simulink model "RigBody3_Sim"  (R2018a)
settings: Solver=ode3  StartTime=0.0  StopTime=5000  FixedStep=Tsr  RelTol=1e-3  EnableMultiTasking=on
InitFcn:
  | run
StopFcn:
  | pl
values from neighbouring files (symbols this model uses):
  d2r = pi/180    (= 0.0174532925199)    [orbitic.m]    (also in Quan.m; run.m; runf.m)
  Int_IC = [qti', 0 0, h0i(1:3)', 0 0, wr0, Vec0'*M0, Pec0']    [run.m]
  Kq1 = I22*ww^2 - 3*wo2*(I11-I33)    [run.m]
  Kq2 = 2*I22*zet*ww    [run.m]
  Kqi = 0.0005    [run.m]
  Kr1 = (0.1*I11*I33*zet^2/Hy0) - sqrt( ((0.01^zet^4*I11^2*I33^2)/Hy0^2)+(4*I11*I33*zet^2) )    [run.m]
  Kr2 = 0.05*Kr1    [run.m]
  Kr3 = 0.04*zet*(Kr2-Hy0) * sqrt(abs(Hy0/(I11*I33)))    [run.m]
  nt = 7    [run.m]    (also in runf.m)
  r2d = 180/pi    (= 57.2957795131)    [pl.m]    (also in pl2.m; run.m; plf.m; runf.m)
  Tmax = 0.05    [run.m]
  Tsr = 0.1    [run.m]
  wo = 0.00113    [run.m]
undefined symbols (not defined in the file or in its folder): DiscIntNeverNeededParam, Mode_Switch, Phase_Plane, RW_Steering, Vehi_3B3W
libraries: simulink x4

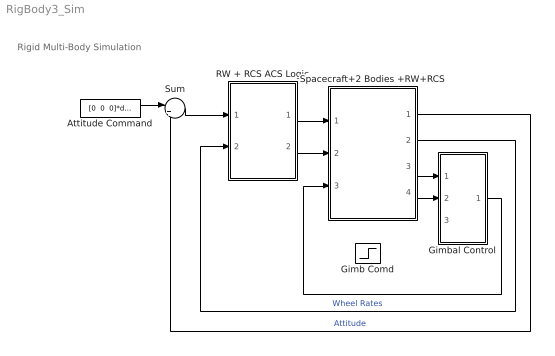
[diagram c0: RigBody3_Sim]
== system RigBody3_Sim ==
  note: Rigid Multi-Body Simulation
  Attitude Command : Constant  Value="[0  0  0]*d2r"
  Gimb Comd : Step  Time=[1, 1]*2000  After=[5, 5]*d2r  SampleTime=0
  Gimbal Control : Subsystem
  RW + RCS ACS Logic : Subsystem
  Spacecraft+2 Bodies +RW+RCS : Subsystem
  Sum : Sum  Inputs=|+-
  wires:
  Spacecraft+2 Bodies +RW+RCS/2(Wrw) -> RW + RCS ACS Logic/2(wr(i))  "Wheel Rates"
  Attitude Command/1 -> Sum/1
  Spacecraft+2 Bodies +RW+RCS/1(att) -> Sum/2  "Attitude"
  Sum/1 -> RW + RCS ACS Logic/1(atter)
  RW + RCS ACS Logic/2(Trwi) -> Spacecraft+2 Bodies +RW+RCS/2(Trw)
  RW + RCS ACS Logic/1(Frcs) -> Spacecraft+2 Bodies +RW+RCS/1(Fjets)
  Spacecraft+2 Bodies +RW+RCS/4(Gmb-dot) -> Gimbal Control/2(Grat)
  Spacecraft+2 Bodies +RW+RCS/3(gimb) -> Gimbal Control/1(Gimb)
  Gimbal Control/1(Trq) -> Spacecraft+2 Bodies +RW+RCS/3(Tgimb)

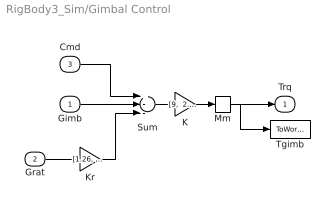
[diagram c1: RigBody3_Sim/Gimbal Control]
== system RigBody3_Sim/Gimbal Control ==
  Gimb : Inport
  Grat : Inport  Port=2
  Cmd : Inport  Port=3
  K : Gain  Gain="[9,  2.85]"
  Kr : Gain  Gain="[1.26,  1.14]"
  Mm : Memory  InheritSampleTime=on
  Sum : Sum  Inputs=+--
  Tgimb : ToWorkspace  VariableName=Tgimb  SampleTime=-1
  Trq : Outport
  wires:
  Sum/1 -> K/1
  Gimb/1 -> Sum/2
  Grat/1 -> Kr/1
  K/1 -> Mm/1
  Kr/1 -> Sum/3
  Cmd/1 -> Sum/1
  Mm/1 -> Trq/1, Tgimb/1

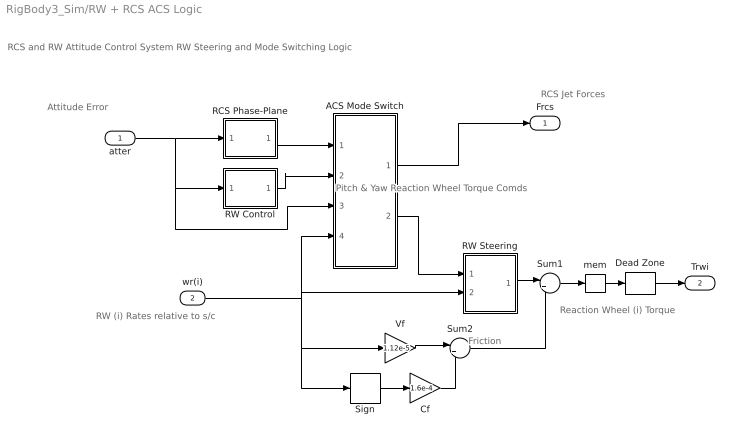
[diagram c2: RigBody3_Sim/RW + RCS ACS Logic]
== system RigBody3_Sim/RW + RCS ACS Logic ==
  note: RCS Jet Forces
  note: RW (i) Rates relative to s/c
  note: Attitude Error
  note: Pitch & Yaw Reaction Wheel Torque Comds
  note: Friction
  note: Reaction Wheel (i) Torque
  note: RCS and RW Attitude Control System RW Steering and Mode Switching Logic
  atter : Inport
  wr(i) : Inport  Port=2
  ACS Mode Switch : Subsystem
  Cf : Gain  Gain=1.6e-4
  Dead Zone : DeadZone  LowerValue=-[1, 1, 1]*Tmax/1000  UpperValue=[1 1 1]*Tmax/1000
  RCS Phase-Plane : Subsystem
  RW Control : Subsystem
  RW Steering : Subsystem
  Sign : Signum
  Sum1 : Sum  Inputs=|+-
  Sum2 : Sum  Inputs=|++
  Vf : Gain  Gain=1.12e-5
  mem : Memory  InheritSampleTime=on
  Frcs : Outport
  Trwi : Outport  Port=2
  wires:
  atter/1 -> RCS Phase-Plane/1(atter), ACS Mode Switch/3(atter), RW Control/1(atti)
  RW Control/1(Tc) -> ACS Mode Switch/2(Trw)
  RCS Phase-Plane/1(f(nt)) -> ACS Mode Switch/1(Frcs)
  ACS Mode Switch/2(" Trw") -> RW Steering/1(Trwc)
  ACS Mode Switch/1(" Frcs") -> Frcs/1
  wr(i)/1 -> Vf/1, Sign/1, RW Steering/2(wr(1)), ACS Mode Switch/4(wr(i))
  Sum2/1 -> Sum1/2
  Sign/1 -> Cf/1
  Vf/1 -> Sum2/1
  Cf/1 -> Sum2/2
  RW Steering/1(Twi) -> Sum1/1
  Sum1/1 -> mem/1
  mem/1 -> Dead Zone/1
  Dead Zone/1 -> Trwi/1

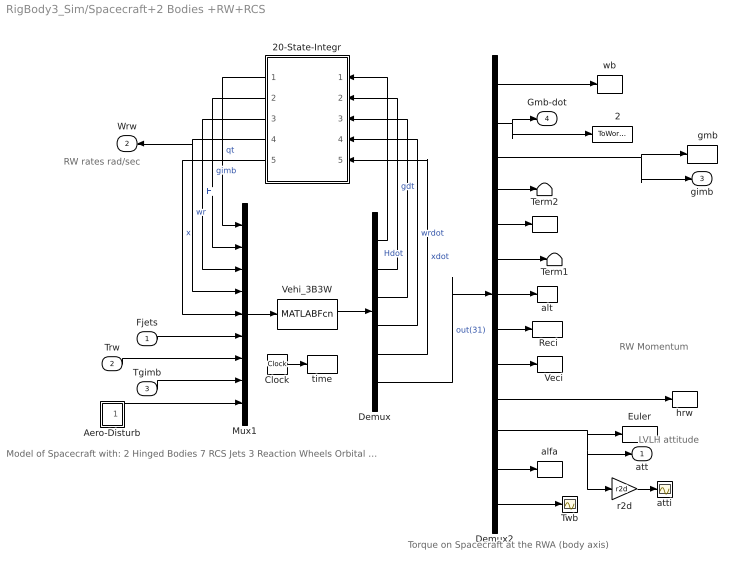
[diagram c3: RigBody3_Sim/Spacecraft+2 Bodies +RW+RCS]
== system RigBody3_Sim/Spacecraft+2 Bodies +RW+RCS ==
  note: RW rates rad/sec
  note: RW Momentum
  note: Model of Spacecraft with: 2 Hinged Bodies 7 RCS Jets 3 Reaction Wheels Orbital Dynamics
  note: LVLH attitude
  note: Torque on Spacecraft at the RWA (body axis)
  Fjets : Inport
  Trw : Inport  Port=2
  Tgimb : Inport  Port=3
  "    " : ToWorkspace  VariableName=hsys  SampleTime=-1
  "    2" : ToWorkspace  VariableName=Gimdot  SampleTime=-1
  "    gmb" : ToWorkspace  VariableName=Gimb  SampleTime=-1
  "   Veci" : ToWorkspace  VariableName=Veci  SampleTime=-1
  "  Reci " : ToWorkspace  VariableName=Reci  SampleTime=-1
  20-State-Integr : Subsystem
  Aero-Disturb : Subsystem
  Clock : Clock
  Demux : Demux  Outputs="[4,2,5,3,6,  31]"
  Demux2 : Demux  Outputs=[3,2,2,1, 3,2, 1,3,3,3,3, 2,3]
  Euler : ToWorkspace  VariableName=Euler  SampleTime=-1
  Mux1 : Mux  Inputs="[4,2,5,3,6,  nt,3,2,3]"
  Term1 : Terminator
  Term2 : Terminator
  Twb : Scope
  Vehi_3B3W : MATLABFcn  MATLABFcn=Vehi_3B3W( u(1:20), u(21:20+nt), u(21+nt:23+nt), u(24+nt:25+nt), u(26+nt:28+nt) )  OutputDimensions=51
  alfa : ToWorkspace  VariableName=alfa  SampleTime=-1
  alt : ToWorkspace  VariableName=alt  SampleTime=-1
  atti : Scope
  hrw : ToWorkspace  VariableName=hrw  SampleTime=-1
  r2d : Gain  Gain=r2d
  time : ToWorkspace  VariableName=time  SampleTime=-1
  wb : ToWorkspace  VariableName=wb  SampleTime=-1
  att : Outport
  Wrw : Outport  Port=2
  gimb : Outport  Port=3
  Gmb-dot : Outport  Port=4
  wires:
  Demux2/9 -> "   Veci"/1
  Vehi_3B3W/1 -> Demux/1
  20-State-Integr/1(qt) -> Mux1/1  "qt"
  20-State-Integr/2(gimb) -> Mux1/2  "gimb"
  20-State-Integr/3(H) -> Mux1/3  "H"
  20-State-Integr/4(wr) -> Wrw/1, Mux1/4  "wr"
  20-State-Integr/5(x) -> Mux1/5  "x"
  Demux/6 -> Demux2/1  "out(31)"
  Demux/1 -> 20-State-Integr/1(qdot)
  Demux/2 -> 20-State-Integr/2(gmbdot)  "gdt"
  Demux/3 -> 20-State-Integr/3(Hdot)  "Hdot"
  Demux/4 -> 20-State-Integr/4(wrdor)  "wrdot"
  Demux/5 -> 20-State-Integr/5(xdot)  "xdot"
  Demux2/12 -> alfa/1
  Demux2/11 -> Euler/1, att/1, r2d/1
  Demux2/10 -> hrw/1
  Demux2/8 -> "  Reci "/1
  Demux2/7 -> alt/1
  Demux2/5 -> "    "/1
  Demux2/6 -> Term1/1
  Demux2/1 -> wb/1
  Demux2/4 -> Term2/1
  Demux2/2 -> Gmb-dot/1, "    2"/1
  Demux2/3 -> gimb/1, "    gmb"/1
  Clock/1 -> time/1
  Tgimb/1 -> Mux1/8
  Aero-Disturb/1(Td) -> Mux1/9
  Trw/1 -> Mux1/7
  Fjets/1 -> Mux1/6
  Mux1/1 -> Vehi_3B3W/1
  r2d/1 -> atti/1
  Demux2/13 -> Twb/1

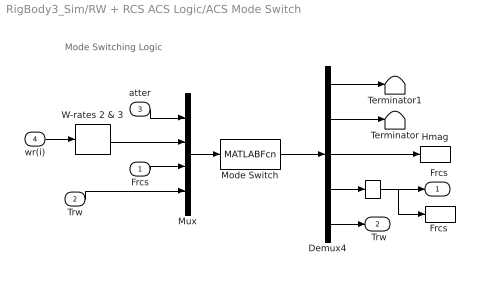
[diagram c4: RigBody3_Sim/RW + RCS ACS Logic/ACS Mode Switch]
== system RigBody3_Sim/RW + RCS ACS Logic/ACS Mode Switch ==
  note: Mode Switching Logic
  Frcs : Inport
  Trw : Inport  Port=2
  atter : Inport  Port=3
  wr(i) : Inport  Port=4
  "   " : Memory
  Demux4 : Demux  Outputs="[1 1 1 nt  2]"
  "Frcs " : ToWorkspace  VariableName=Frcs  SampleTime=-1
  Hmag : ToWorkspace  VariableName=Hmag  SampleTime=-1
  Mode Switch : MATLABFcn  MATLABFcn=Mode_Switch( u(1:3), u(4:5), u(6:5+nt), u(6+nt:7+nt) )  OutputDimensions=3+nt+2
  Mux : Mux  Inputs="[3  2  nt 2]"
  Terminator : Terminator
  Terminator1 : Terminator
  W-rates 2 & 3 : Selector  InputPortWidth=3  IndexOptions=Index vector (dialog)  Indices="[2  3]"  OutputSizes=1
  " Frcs" : Outport
  " Trw" : Outport  Port=2
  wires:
  Demux4/3 -> Hmag/1
  Demux4/2 -> Terminator/1
  Demux4/1 -> Terminator1/1
  W-rates 2 & 3/1 -> Mux/2
  "   "/1 -> " Frcs"/1, "Frcs "/1
  Demux4/5 -> " Trw"/1
  Demux4/4 -> "   "/1
  Mode Switch/1 -> Demux4/1
  Trw/1 -> Mux/4
  Frcs/1 -> Mux/3
  wr(i)/1 -> W-rates 2 & 3/1
  Mux/1 -> Mode Switch/1
  atter/1 -> Mux/1

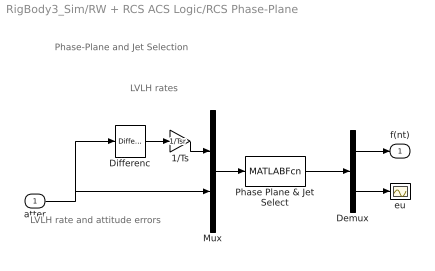
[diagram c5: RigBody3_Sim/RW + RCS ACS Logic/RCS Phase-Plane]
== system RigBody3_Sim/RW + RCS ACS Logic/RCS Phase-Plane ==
  note: Phase-Plane and Jet Selection
  note: LVLH rate and attitude errors
  note: LVLH rates
  atter : Inport
  1/Ts : Gain  Gain=1/Tsr
  Demux : Demux  Outputs=[nt, 3]
  Differenc : simulink/Discrete/Difference  ICPrevInput=0.0  InputProcessing=Inherited  OutMin=[]  OutMax=[]  OutDataType=sfix(16)  OutScaling=2^-10  DoSatur=off
  Mux : Mux  Inputs="[3  3]"
  Phase Plane & Jet Select : MATLABFcn  MATLABFcn=Phase_Plane( u(1:3), u(4:6) )  OutputDimensions=nt + 3
  eu : Scope
  f(nt) : Outport
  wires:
  atter/1 -> Mux/2, Differenc/1
  1/Ts/1 -> Mux/1
  Demux/2 -> eu/1
  Demux/1 -> f(nt)/1
  Phase Plane & Jet Select/1 -> Demux/1
  Mux/1 -> Phase Plane & Jet Select/1
  Differenc/1 -> 1/Ts/1

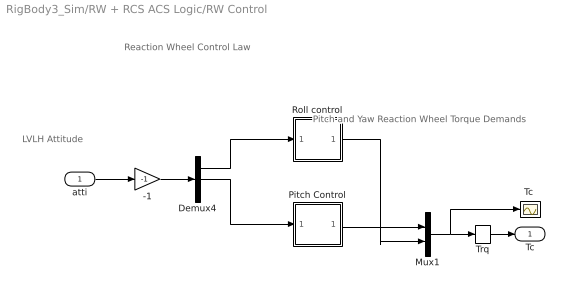
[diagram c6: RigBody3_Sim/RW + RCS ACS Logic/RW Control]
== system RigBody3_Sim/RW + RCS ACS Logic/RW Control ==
  note: Pitch and Yaw Reaction Wheel Torque Demands
  note: LVLH Attitude
  note: Reaction Wheel Control Law
  atti : Inport
  -1 : Gain  Gain=-1
  Demux4 : Demux  Outputs=3
  Mux1 : Mux  Inputs=2
  Pitch Control : Subsystem
  Roll control : Subsystem
  "Tc " : Scope
  Trq : Memory
  Tc : Outport
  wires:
  Demux4/1 -> Roll control/1(phi)
  Pitch Control/1(Tcy) -> Mux1/1
  Demux4/2 -> Pitch Control/1(the)
  atti/1 -> -1/1
  Mux1/1 -> Trq/1, "Tc "/1
  -1/1 -> Demux4/1
  Roll control/1(Tcz) -> Mux1/2
  Trq/1 -> Tc/1

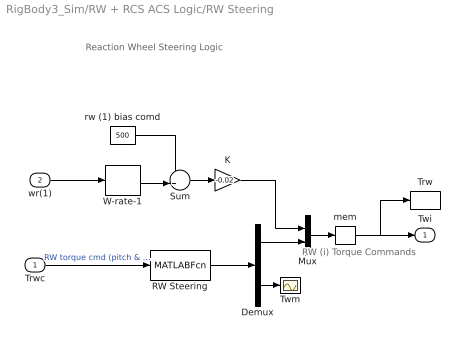
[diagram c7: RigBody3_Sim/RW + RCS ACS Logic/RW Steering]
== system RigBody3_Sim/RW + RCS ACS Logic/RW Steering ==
  note: RW (i) Torque Commands
  note: Reaction Wheel Steering Logic
  Trwc : Inport
  wr(1) : Inport  Port=2
  Demux : Demux  Outputs=[2, 1]
  K : Gain  Gain=-0.02
  Mux : Mux  Inputs=[1,2]
  RW Steering : MATLABFcn  MATLABFcn=RW_Steering( u(1:2) )  OutputDimensions=3
  Sum : Sum  Inputs=++|
  Trw : ToWorkspace  VariableName=Trw  SampleTime=-1
  Twm : Scope
  W-rate-1 : Selector  InputPortWidth=3  IndexOptions=Index vector (dialog)  Indices=[1]  OutputSizes=1
  mem : Memory
  rw (1) bias comd : Constant  Value=500
  Twi : Outport
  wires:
  Demux/2 -> Twm/1
  Demux/1 -> Mux/2
  RW Steering/1 -> Demux/1
  Trwc/1 -> RW Steering/1  "RW torque cmd (pitch & yaw)"
  Mux/1 -> mem/1
  wr(1)/1 -> W-rate-1/1
  Sum/1 -> K/1
  rw (1) bias comd/1 -> Sum/1
  W-rate-1/1 -> Sum/2
  K/1 -> Mux/1
  mem/1 -> Twi/1, Trw/1

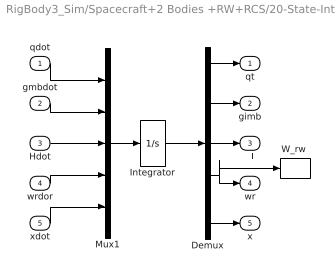
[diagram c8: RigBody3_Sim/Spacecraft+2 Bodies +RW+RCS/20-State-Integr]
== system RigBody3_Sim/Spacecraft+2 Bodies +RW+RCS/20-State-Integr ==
  qdot : Inport
  gmbdot : Inport  Port=2
  Hdot : Inport  Port=3
  wrdor : Inport  Port=4
  xdot : Inport  Port=5
  Demux : Demux  Outputs=[4,2,5,3,6]
  Integrator : Integrator  InitialCondition=Int_IC
  Mux1 : Mux  Inputs=[4,2,5,3,6]
  "W_rw " : ToWorkspace  VariableName=W_rw  SampleTime=-1
  qt : Outport
  gimb : Outport  Port=2
  H : Outport  Port=3
  wr : Outport  Port=4
  x : Outport  Port=5
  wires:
  Mux1/1 -> Integrator/1
  Integrator/1 -> Demux/1
  qdot/1 -> Mux1/1
  gmbdot/1 -> Mux1/2
  Hdot/1 -> Mux1/3
  wrdor/1 -> Mux1/4
  xdot/1 -> Mux1/5
  Demux/1 -> qt/1
  Demux/2 -> gimb/1
  Demux/3 -> H/1
  Demux/4 -> "W_rw "/1, wr/1
  Demux/5 -> x/1

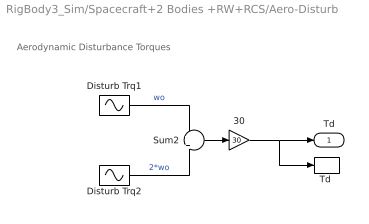
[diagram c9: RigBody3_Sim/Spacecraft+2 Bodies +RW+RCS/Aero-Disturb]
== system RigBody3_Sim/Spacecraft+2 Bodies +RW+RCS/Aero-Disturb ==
  note: Aerodynamic Disturbance Torques
  30 : Gain  Gain=30
  Disturb Trq1 : Sin  Amplitude="[0.0,   1,   0.2]*0.0001"  Bias="[0.0,  0.5,  0.15]*0.0001"  Frequency=[wo, wo, wo]  SampleTime=0
  Disturb Trq2 : Sin  Amplitude=[0, 1.2, 1]*0.0001  Bias=[0 0 0]  Frequency=[wo, wo, wo]*2  SampleTime=0
  Sum2 : Sum  Inputs=+|+
  "Td " : ToWorkspace  VariableName=Td  SampleTime=-1
  Td : Outport
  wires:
  30/1 -> "Td "/1, Td/1
  Disturb Trq2/1 -> Sum2/2  "2*wo"
  Sum2/1 -> 30/1
  Disturb Trq1/1 -> Sum2/1  "wo"

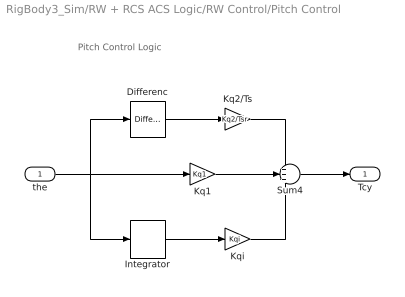
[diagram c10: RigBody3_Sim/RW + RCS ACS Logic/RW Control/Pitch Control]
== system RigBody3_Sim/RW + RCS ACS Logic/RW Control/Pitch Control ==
  note: Pitch Control Logic
  the : Inport
  Differenc : simulink/Discrete/Difference  ICPrevInput=0.0  InputProcessing=Inherited  OutMin=[]  OutMax=[]  OutDataType=sfix(16)  OutScaling=2^-10  DoSatur=off
  Integrator : DiscreteIntegrator  SampleTime=Tsr  ICPrevOutput=DiscIntNeverNeededParam  ICPrevScaledInput=DiscIntNeverNeededParam
  Kq1 : Gain  Gain=Kq1
  Kq2/Ts : Gain  Gain=Kq2/Tsr
  Kqi : Gain  Gain=Kqi
  Sum4 : Sum  Inputs=+++
  Tcy : Outport
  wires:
  Kq1/1 -> Sum4/2
  Sum4/1 -> Tcy/1
  Kq2/Ts/1 -> Sum4/1
  the/1 -> Kq1/1, Integrator/1, Differenc/1
  Kqi/1 -> Sum4/3
  Integrator/1 -> Kqi/1
  Differenc/1 -> Kq2/Ts/1

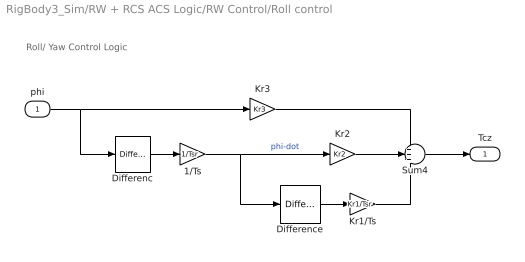
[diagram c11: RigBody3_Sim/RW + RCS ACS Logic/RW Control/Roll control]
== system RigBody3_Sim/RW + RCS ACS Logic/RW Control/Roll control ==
  note: Roll/ Yaw Control Logic
  phi : Inport
  1/Ts : Gain  Gain=1/Tsr
  Differenc : simulink/Discrete/Difference  ICPrevInput=0.0  InputProcessing=Inherited  OutMin=[]  OutMax=[]  OutDataType=sfix(16)  OutScaling=2^-10  DoSatur=off
  Difference : simulink/Discrete/Difference  ICPrevInput=0.0  InputProcessing=Inherited  OutMin=[]  OutMax=[]  OutDataType=sfix(16)  OutScaling=2^-10  DoSatur=off
  Kr1/Ts : Gain  Gain=Kr1/Tsr
  Kr2 : Gain  Gain=Kr2
  Kr3 : Gain  Gain=Kr3
  Sum4 : Sum  Inputs=+++
  Tcz : Outport
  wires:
  Kr3/1 -> Sum4/1
  Kr2/1 -> Sum4/2
  Kr1/Ts/1 -> Sum4/3
  phi/1 -> Kr3/1, Differenc/1
  Sum4/1 -> Tcz/1
  Difference/1 -> Kr1/Ts/1
  Differenc/1 -> 1/Ts/1
  1/Ts/1 -> Kr2/1, Difference/1  "phi-dot"
